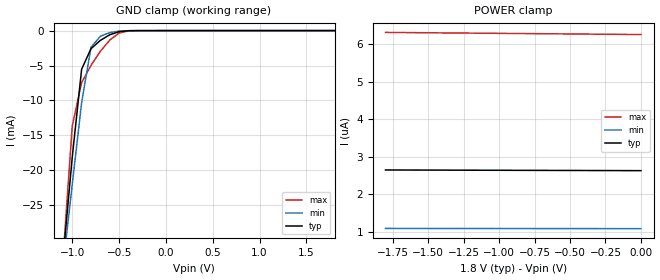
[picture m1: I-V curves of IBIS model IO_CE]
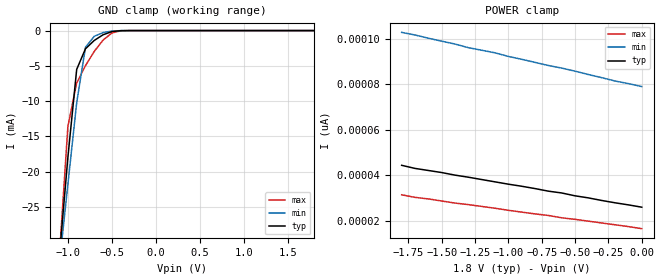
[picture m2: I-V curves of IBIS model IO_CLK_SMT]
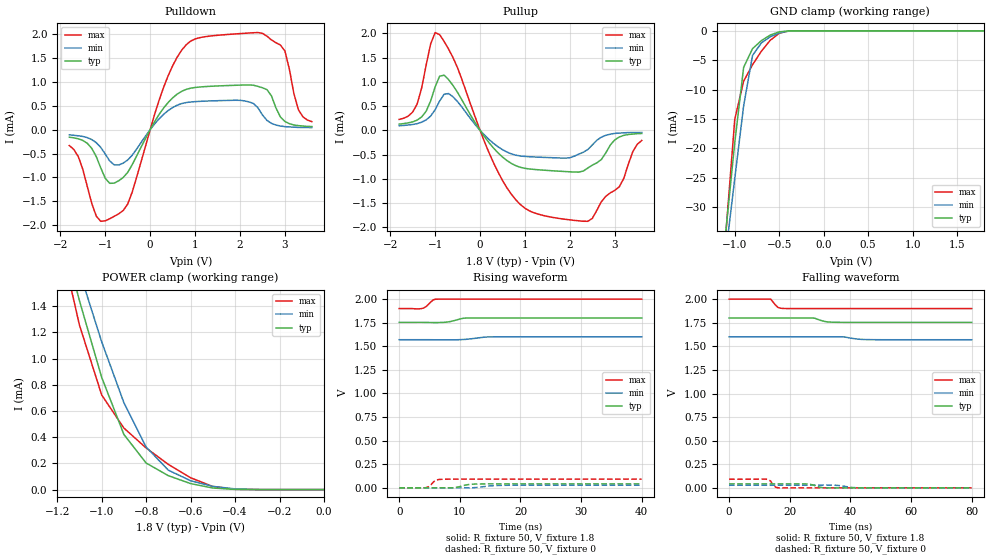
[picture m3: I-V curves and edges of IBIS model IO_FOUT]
[IBIS Ver]   3.2
[Comment Char]   |_char
[File name]   rx8803sa_18.ibs
[File Rev]   1.0
[Date]   Jan 16, 2013
[Source]   This file orginated at SEIKO EPSON Corp.
[Copyright]
   Copyright 2013, SEIKO EPSON Corp.
[Component]   8803sa_18
[Manufacturer]  SEIKO EPSON Corp.
[Package]
| variable   typ   min   max
R_pkg   3.00m   NA   NA
L_pkg   3.70nH   NA   NA
C_pkg   0.70pF   NA   NA
[Pin] signal_name   model_name
1   CE   IO_CE
2   SCL   IO_CLK_SMT
3   FOUT   IO_FOUT
4   NC   NC
|5   TEST   IO_TEST
6   VDD   POWER
7   FOE   IO_FOE
8   NC   NC
9   EVIN   IO_STAMP
10   /INT   IO_IRQ
11   VSS   GND
12   T2(VPP)   POWER
13   SDA   IO_DIO_SMT
14   NC   NC
| Models and submodels in the file (9): IO_CE (Input), IO_CLK_SMT (Input), IO_FOUT (3-state), IO_TEST (Input), IO_FOE (Input), IO_STAMP (Input), IO_IRQ (Open_drain), IO_DIO_SMT (I/O_open_drain), IO_IN (Input)
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[Model]   IO_CE
Model_type Input
Enable Active-Low
Polarity Non-Inverting
Vinh=1.44
Vinl=0.36
C_comp   5p   4p   6p
[Temperature Range] 25   85   -40
[Voltage Range]   1.8   1.6   2.0
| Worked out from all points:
|   GND clamp passes 1 mA (typ) near -0.65 V on its own axis
[GND Clamp]
-1.8V     -138.9mA   -119.4mA   -172.4mA
-1.1V     -32.77mA   -33.87mA   -32.85mA
-1V       -18.1mA    -22.01mA   -13.64mA
-900mV    -5.528mA   -10.31mA   -7.436mA
-800mV    -2.584mA   -2.379mA   -4.976mA
-700mV    -1.397mA   -811.7uA   -2.953mA
-600mV    -595.6uA   -284.2uA   -1.355mA
-500mV    -148uA     -63.68uA   -350.4uA
-400mV    -17.85uA   -8.651uA   -34uA
1.8V      2.629uA    1.081uA    6.256uA
[POWER Clamp]
-1.8V     2.647uA    1.087uA    6.32uA
-1.4V     2.643uA    1.085uA    6.307uA
-400mV    2.633uA    1.082uA    6.275uA
0V        2.629uA    1.081uA    6.262uA
[Model]   IO_CLK_SMT
Model_type Input
Enable Active-Low
Polarity Non-Inverting
Vinh=1.44
Vinl=0.36
C_comp   5p   4p   6p
[Temperature Range] 25   85   -40
[Voltage Range]   1.8   1.6   2.0
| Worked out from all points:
|   GND clamp passes 1 mA (typ) near -0.65 V on its own axis
[GND Clamp]
-1.8V     -136.6mA   -117.3mA   -169.7mA
-1.1V     -32.43mA   -33.46mA   -32.61mA
-1V       -17.96mA   -21.79mA   -13.59mA
-900mV    -5.499mA   -10.22mA   -7.421mA
-800mV    -2.576mA   -2.362mA   -4.965mA
-700mV    -1.392mA   -807.3uA   -2.943mA
-600mV    -591.5uA   -281.9uA   -1.347mA
-500mV    -144.6uA   -61.93uA   -343.6uA
-400mV    -15.25uA   -7.313uA   -28.72uA
1.8V      25.81pA    81.4pA     14.78pA
[POWER Clamp]
-1.8V     44.34pA    102.8pA    31.38pA
-1.7V     42.97pA    101.6pA    30.24pA
-1.5V     41.15pA    98.91pA    28.65pA
-1.4V     40.02pA    97.66pA    27.74pA
-1.3V     39.11pA    96.07pA    27.06pA
-1.1V     37.06pA    93.79pA    25.47pA
-1V       36.04pA    92.2pA     24.56pA
-700mV    32.97pA    88.22pA    22.28pA
-600mV    32.17pA    87.08pA    21.26pA
-500mV    30.92pA    85.72pA    20.58pA
-200mV    27.85pA    81.4pA     18.19pA
0V        25.92pA    78.96pA    16.48pA
[Model]   IO_FOUT
Model_type 3-state
Enable Active-High
Polarity Non-Inverting
Vmeas=0.90
C_comp   5p   4p   6p
[Temperature Range] 25   85   -40
[Voltage Range]   1.8   1.6   2.0
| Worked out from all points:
|   slope of the pulldown table from 0 to 0.27 V, typ, clamps not added: 657 ohm
|   slope of the pullup table from 0 to 0.27 V, typ, clamps not added: 810 ohm
|   GND clamp passes 1 mA (typ) near -0.63 V on its own axis
|   POWER clamp passes 1 mA (typ) near -1.02 V on its own axis
[Pullup]
-1.8V     128.3uA    93.14uA    224.4uA
-1.4V     209.8uA    136.8uA    542.3uA
-1.2V     393.9uA    214.9uA    1.345mA
-1V       896.8uA    423.3uA    2.016mA
-900mV    1.116mA    603.3uA    1.974mA
-700mV    1.044mA    758.4uA    1.674mA
400mV     -465.3uA   -340.2uA   -860.9uA
1.1V      -798.2uA   -545.4uA   -1.663mA
2.4V      -778.2uA   -395.9uA   -1.878mA
3.1V      -138.4uA   -57.99uA   -1.166mA
3.4V      -77.85uA   -45.23uA   -442.5uA
3.6V      -65.98uA   -45.18uA   -210.1uA
[Pulldown]
-1.8V     -158.4uA   -110.1uA   -332.8uA
-1.6V     -192.5uA   -129.6uA   -564.3uA
-1.2V     -564.3uA   -272.7uA   -1.807mA
-900mV    -1.122mA   -655uA     -1.861mA
-600mV    -999.6uA   -699.4uA   -1.689mA
500mV     662.2uA    460.7uA    1.332mA
1.4V      907.4uA    600.8uA    1.96mA
2.3V      926.3uA    545.6uA    2.023mA
2.6V      834.8uA    192uA      1.951mA
2.9V      263.3uA    74.61uA    1.766mA
3.3V      83.32uA    45.86uA    415.9uA
3.6V      63.61uA    42.32uA    166.2uA
[GND Clamp]
-1.8V     -143.3mA   -129.1mA   -177.3mA
-1.1V     -34.07mA   -37.78mA   -34.52mA
-1V       -19.07mA   -25.17mA   -15.1mA
-900mV    -6.217mA   -12.77mA   -8.569mA
-800mV    -3.038mA   -4.193mA   -5.779mA
-700mV    -1.663mA   -2.048mA   -3.456mA
-600mV    -716.1uA   -1.013mA   -1.603mA
-500mV    -178.4uA   -369.5uA   -418.8uA
-400mV    -19.08uA   -74.17uA   -35.91uA
1.8V      42.86pA    91.89nA    26.26pA
[POWER Clamp]
-1.8V     6.534mA    6.037mA    7.441mA
-1.2V     2.101mA    2.242mA    2.001mA
-1.1V     1.442mA    1.665mA    1.256mA
-1V       856.8uA    1.128mA    722.6uA
-900mV    420.7uA    663uA      469.5uA
-800mV    202.7uA    324.8uA    317.8uA
-700mV    106.2uA    148.3uA    192.1uA
-600mV    46.01uA    67.69uA    90.33uA
-500mV    12.08uA    24.6uA     23.88uA
-400mV    1.58uA     5.546uA    2.09uA
0V        42.97pA    999pA      31.6pA
[Falling Waveform]
R_fixture=50
V_fixture=1.8
V_fixture_min=1.6
V_fixture_max=2.0
0s        1.8V       1.6V       2V
13.74ns   1.8V       1.6V       2V
16.16ns   1.8V       1.6V       1.912V
17.78ns   1.8V       1.6V       1.902V
27.47ns   1.8V       1.6V       1.9V
31.52ns   1.764V     1.6V       1.9V
34.75ns   1.755V     1.6V       1.9V
37.98ns   1.754V     1.599V     1.9V
46.06ns   1.754V     1.571V     1.9V
80ns      1.754V     1.57V      1.9V
[Falling Waveform]
R_fixture=50
V_fixture=0
V_fixture_min=0
V_fixture_max=0
0s        42.18mV    28.22mV    91.9mV
12.93ns   42.17mV    28.22mV    88.16mV
13.74ns   42.18mV    28.22mV    70.45mV
14.55ns   42.18mV    28.22mV    29.96mV
15.35ns   42.18mV    28.22mV    7.996mV
16.16ns   42.19mV    28.22mV    359.9uV
25.86ns   41.09mV    28.28mV    9.452uV
31.52ns   485.5uV    28.63mV    -18.42uV
42.83ns   -7.067uV   210.4uV    4.316uV
80ns      8.506uV    10.94uV    10.59uV
[Rising Waveform]
R_fixture=50
V_fixture=1.8
V_fixture_min=1.6
V_fixture_max=2.0
0s        1.754V     1.57V      1.9V
3.636ns   1.754V     1.57V      1.899V
4.04ns    1.754V     1.57V      1.906V
4.444ns   1.753V     1.57V      1.922V
5.657ns   1.752V     1.569V     1.994V
6.061ns   1.751V     1.569V     1.999V
8.081ns   1.759V     1.568V     2V
10.91ns   1.799V     1.573V     2V
14.95ns   1.8V       1.6V       2V
40ns      1.8V       1.6V       2V
[Rising Waveform]
R_fixture=50
V_fixture=0
V_fixture_min=0
V_fixture_max=0
0s        0V         0V         0V
4.444ns   29.83uV    -1.196uV   2.236mV
4.848ns   25.64uV    12.76uV    12mV
6.061ns   11.4uV     20.85uV    80.75mV
7.273ns   -102.3uV   15.56uV    91.01mV
8.889ns   472.6uV    -10.07uV   91.83mV
11.31ns   33.37mV    -308.3uV   91.91mV
13.33ns   41.12mV    7.646mV    91.91mV
17.78ns   42.15mV    27.14mV    91.89mV
40ns      42.16mV    28.22mV    91.89mV
[Ramp]
R_load=50
dV/dt_r   2.530E-2/1.670E-9   1.693E-2/2.419E-9   5.513E-2/8.848E-10
dV/dt_f   2.763E-2/2.746E-9   1.817E-2/3.816E-9   5.996E-2/1.492E-9
|[End   IO_FOUT
